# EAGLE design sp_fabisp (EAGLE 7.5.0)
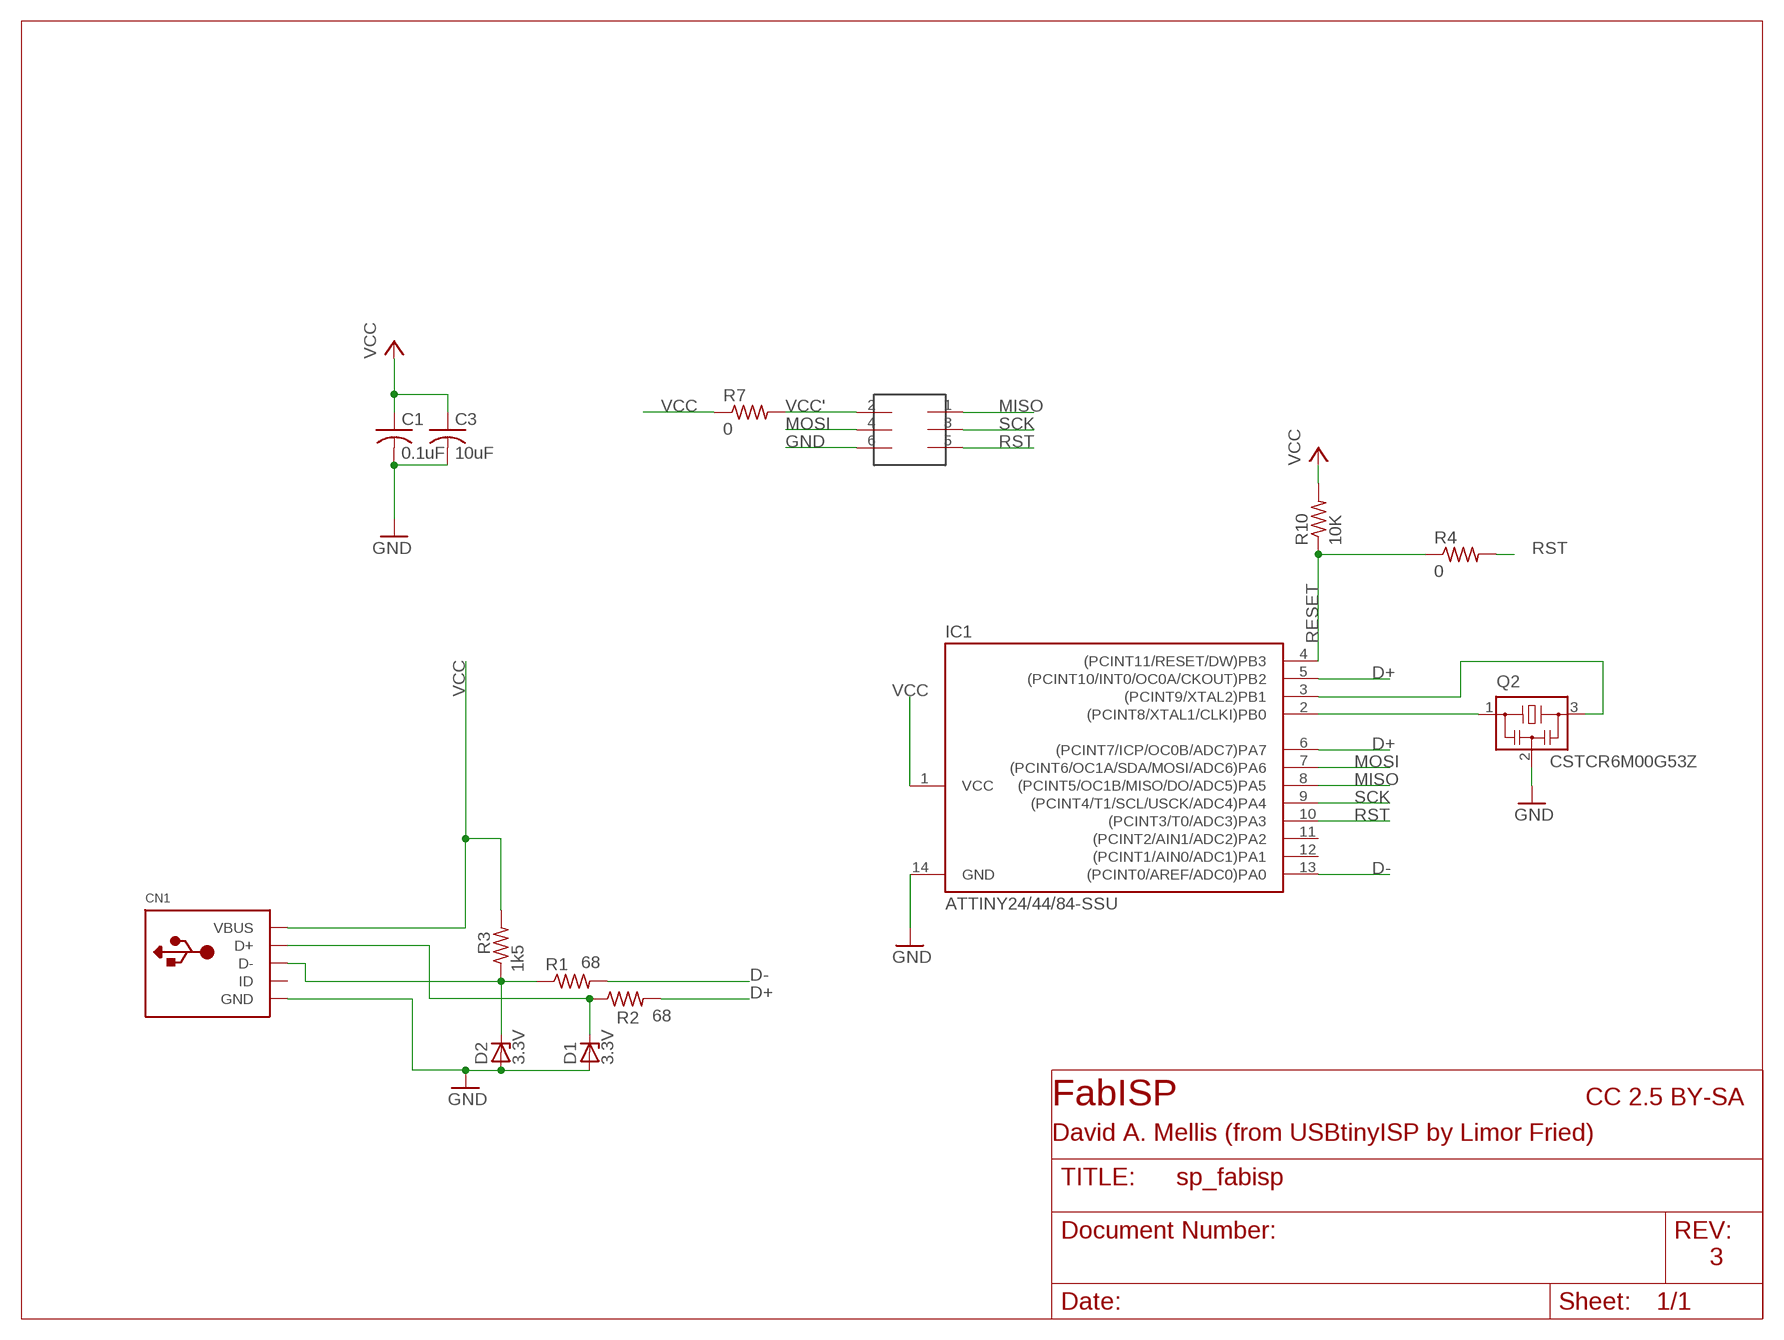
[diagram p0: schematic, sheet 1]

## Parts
C1  0.1uF  C-USC1206  [C1206]
C3  10uF  C-USC1206  [C1206]
CN1  USBMINIB  [USB-MINIB]
D1  3.3V  ZENER_DIODESOD123  [SOD123]
D2  3.3V  ZENER_DIODESOD123  [SOD123]
IC1  ATTINY24/44/84-SSU  [SOIC14]
Q2  CSTCR6M00G53Z  [CSTCR6M]
R1  68  R-US_R1206  [R1206]
R2  68  R-US_R1206  [R1206]
R3  1k5  R-US_R1206  [R1206]
R4  0  R-US_R1206  [R1206]
R7  0  R-US_R1206  [R1206]
R10  10K  R-US_R1206  [R1206]
U$1  2X3HEADER  [2X3_SMD]

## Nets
D+: IC1.5((PCINT10/INT0/OC0A/CKOUT)PB2) IC1.6((PCINT7/ICP/OC0B/ADC7)PA7) R2.2
D-: IC1.13((PCINT0/AREF/ADC0)PA0) R1.2
D_+: CN1.D+ D1.CATHODE R2.1
D_-: CN1.D- D2.CATHODE R1.1 R3.1
GND: C1.2 C3.2 CN1.GND D1.ANODE D2.ANODE IC1.14(GND) Q2.2 U$1.6
MISO: IC1.8((PCINT5/OC1B/MISO/DO/ADC5)PA5) U$1.1
MOSI: IC1.7((PCINT6/OC1A/SDA/MOSI/ADC6)PA6) U$1.4
N$4: IC1.2((PCINT8/XTAL1/CLKI)PB0) Q2.1
N$5: IC1.3((PCINT9/XTAL2)PB1) Q2.3
RESET: IC1.4((PCINT11/RESET/DW)PB3) R4.1 R10.1
RST: IC1.10((PCINT3/T0/ADC3)PA3) R4.2 U$1.5
SCK: IC1.9((PCINT4/T1/SCL/USCK/ADC4)PA4) U$1.3
VCC: C1.1 C3.1 CN1.VBUS IC1.1(VCC) R3.2 R7.1 R10.2
VCC': R7.2 U$1.2
Unconnected: CN1.ID IC1.11((PCINT2/AIN1/ADC2)PA2) IC1.12((PCINT1/AIN0/ADC1)PA1)

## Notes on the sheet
- FabISP | CC 2.5 BY-SA
- David A. Mellis (from USBtinyISP by Limor Fried)
- 3

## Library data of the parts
C1 = rcl-ez:C-US: CAPACITOR, American symbol
C3 = rcl:C-US: CAPACITOR, American symbol
CN1 = adafruit:USB: USB Connectors USBMINIB - Surface Mount Female Mini-B USB Connector 4UConnector: 06564 By microbuilder.eu Thru-hole RA Female Mini-B USB Connector 4UConnector: 18732 By ladyada.net
D1 D2 = ng:ZENER_DIODE: zener diode
IC1 = attiny24_44_84:ATTINY24/44/84
Q2 = FablabTorino:CSTCR: Resonator Source: murata.co.jp; MPN: CSTCR6M00G53-R0; OC_FARNELL: 1170434; OC_NEWARK: 25M8759
R1-R3 R10 = rcl-ez:R-US_: RESISTOR, American symbol
R4 R7 = rcl:R-US_: RESISTOR, American symbol
U$1 = mellis:2X3HEADER

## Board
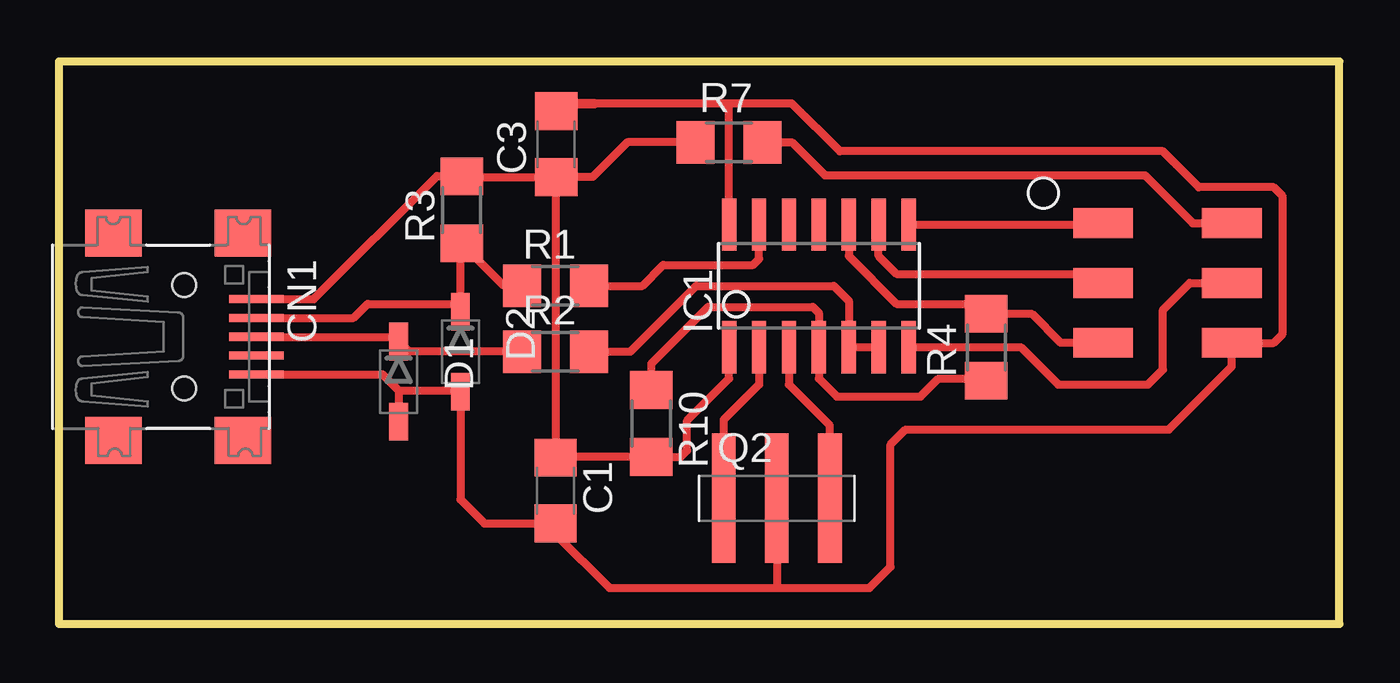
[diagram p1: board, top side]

Size 54.41 x 23.99 mm. Coordinates in mm from the lower left corner, seen from the top.
Outline: 0,0 54.41,0 54.41,23.99 0,23.99 0,0
Copper layers (1*16): Top 0.035mm / dielectric 1.5mm / Bottom 0.035mm
Design rules "default *": minimum track width 10mil, minimum drill 24mil, track to track 16mil, track to pad 16mil, pad to pad 16mil, via to via 16mil, smd to smd 16mil, copper to edge 40mil, drill to drill 8mil, minimum pad ring 10mil, minimum via ring 8mil, stop-mask expansion 4mil, vias tented up to drill 0mil, thermal gap 10mil
Milling: 4 lines

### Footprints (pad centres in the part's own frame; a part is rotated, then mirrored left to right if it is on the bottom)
C1206 = smd 1.6 x 1.8: 1 -1.4,0; 2 1.4,0
USB-MINIB = smd 0.348 x 2.308: D+ 0,4.064; D- -0.8,4.064; GND 1.6,4.064; ID 0.8,4.064; VBUS -1.6,4.064 | smd 2 x 2.4: GND1 -4.4,-2; GND2 -4.4,3.5; GND3 4.4,3.5; GND4 4.4,-2 | hole 1: -2.2,1; 2.2,1
SOD123 = smd 1.6 x 0.8: ANODE 1.7,0; CATHODE -1.7,0
SOIC14 = smd 0.61 x 2.21: 1 -3.81,-2.603; 2 -2.54,-2.603; 3 -1.27,-2.603; 4 0,-2.603; 5 1.27,-2.603; 6 2.54,-2.603; 7 3.81,-2.603; 8 3.81,2.603; 9 2.54,2.603; 10 1.27,2.603; 11 0,2.603; 12 -1.27,2.603; 13 -2.54,2.603; 14 -3.81,2.603
CSTCR6M = smd 1 x 5.5: 1 -2.25,0; 2 0,0; 3 2.25,0
R1206 = smd 1.6 x 1.803: 1 -1.422,0; 2 1.422,0
2X3_SMD = smd 2.54 x 1.27: 1 -2.54,2.54; 2 2.92,2.54; 3 -2.54,0; 4 2.92,0; 5 -2.54,-2.54; 6 2.92,-2.54

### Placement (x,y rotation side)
C1  21.08,5.66 270 top
C3  21.11,20.37 90 top
CN1  4.32,12.19 270 top
D1  14.43,10.29 270 top
D2  17.04,11.56 270 top
IC1  32.26,14.35 0 top
Q2  30.48,5.33 0 top
R1  21.08,14.35 0 top
R2  21.08,11.56 0 top
R3  17.09,17.58 90 top
R4  39.37,11.75 90 top
R7  28.45,20.45 0 top
R10  25.15,8.51 270 top
U$1  46.86,14.48 0 top

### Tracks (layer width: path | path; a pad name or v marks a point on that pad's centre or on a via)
D+
  Top 0.35: IC1.6 IC1.5 33.53,13.72 32.89,14.35 27.05,14.35 24.26,11.56 R2.2
D-
  Top 0.35: R1.2 24.77,14.35 25.65,15.24 29.46,15.24 29.72,15.49 IC1.13
D_+
  Top 0.35: R2.1 14.86,11.56 D1.CATHODE 14.22,12.19 CN1.D+
D_-
  Top 0.35: R1.1 18.9,14.35 R3.1 17.04,16.1 D2.CATHODE 16.71,13.59 13.11,13.59 12.51,12.99 CN1.D-
GND
  Top 0.35: IC1.14 28.45,22.1 | 30.48,1.52 23.37,1.52 21.08,3.81 C1.2 18.06,4.27 17.04,5.28 D2.ANODE 16.99,9.91 14.43,9.91 | 30.48,1.52 34.42,1.52 35.31,2.41 35.31,7.62 35.94,8.26 47.12,8.26 49.78,10.92 U$1.6 51.56,11.94 51.94,12.32 51.94,18.16 51.56,18.54 48.39,18.54 46.86,20.07 33.15,20.07 31.11,22.1 28.45,22.1 | Q2.2 30.48,1.52 | 28.45,22.1 22.73,22.1 | CN1.GND 13.74,10.59 14.43,9.91 | 14.43,9.91 D1.ANODE | 21.43,22.1 C3.2
  Top 0.406: 22.73,22.1 21.43,22.1
MISO
  Top 0.35: IC1.8 44.26,16.95 U$1.1
MOSI
  Top 0.35: IC1.7 40.83,11.75 42.42,10.16 46.23,10.16 46.86,10.79 46.86,13.34 48.01,14.48 U$1.4
N$4
  Top 0.35: IC1.2 29.72,10.16 28.23,8.67 Q2.1
N$5
  Top 0.35: IC1.3 30.99,10.16 32.73,8.42 Q2.3
RESET
  Top 0.35: R4.1 39.34,10.41 37.34,10.41 36.58,9.65 33.02,9.65 32.26,10.41 IC1.4 32.26,13.21 32,13.46 27.56,13.46 25.15,11.05 R10.1
RST
  Top 0.35: IC1.10 33.53,15.62 35.56,13.59 39.01,13.59 R4.2 39.38,13.16 41.31,13.16 42.53,11.94 U$1.5
SCK
  Top 0.35: IC1.9 34.8,15.62 35.56,14.86 43.94,14.86 U$1.3
VCC
  Top 0.35: 21.08,18.95 C1.1 21.11,7.09 R10.2 26.39,7.09 26.67,7.37 26.67,8.64 28.45,10.41 IC1.1 | R7.1 24.13,20.45 22.66,18.97 C3.1 21.08,18.95 | 21.08,18.95 17.15,18.95 R3.2 17.07,19.02 16.05,19.02 10.82,13.79 CN1.VBUS
VCC'
  Top 0.35: U$1.2 48.13,17.02 46.1,19.05 32.51,19.05 31.11,20.45 R7.2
